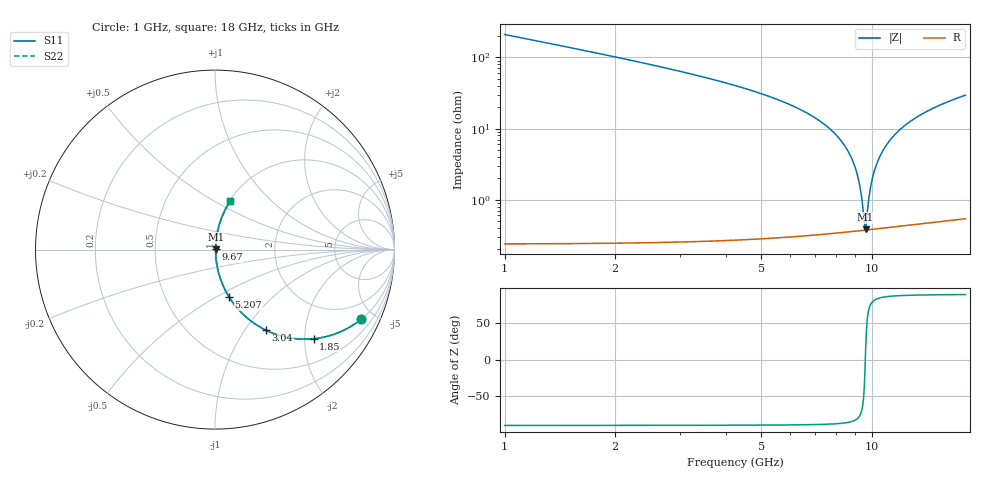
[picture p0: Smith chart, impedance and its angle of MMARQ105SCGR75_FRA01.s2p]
! MMARQ105SCGR75_FRA01  S-PARAMETER MODEL  ( General Type )
! Model Generated by TAIYO YUDEN Corporation (http://www.ty-top.com)
! Version 1.0
! TAIYO YUDEN Control No. 200326
! Copyright(c) 2020 TAIYO YUDEN CO.,LTD. All Rights Reserved.
! Product Description (link to TY-COMPAS)
! https://ds.yuden.co.jp/TYCOMPAS/or/detail?pn=MMARQ105SCGR75BFRA01&u=M
! Products Name : Multilayer Ceramic Capacitors
! Characteristics :
!  Capacitance : 0.75 pF , Rated Voltage : 250V , TCC : CG / C0G
!  Case Size : 1.0 x 0.5 / 0.039 x 0.02 [mm/inch] , Thickness : 0.5 / 0.02 [mm/inch]
!  (Conditions: Temperature = 25 degC , DC Bias Current/Voltage = 0A / 0V)
! External Node Assignments :
!  1  o---| |---o  2
! GND o---------o GND
! Frequency Range : 1GHz  -  18GHz  [ 401 STEP ]
# MHz S RI R 50
! Freq[MHz].  S11 Real  S11 Imag  S21 Real  S21 Imag  S12 Real  S12 Imag  S22 Real  S22 Imag
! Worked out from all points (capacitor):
!   401 points, 1 GHz to 18 GHz, reference 50 ohm
!   read as one part in series: C = 750 fF near 1.085 GHz
!   lowest |Z| = 384 mohm at 9.627 GHz (marker M1)
!   series resonance near 9.608 GHz, so ESL is about 370 pH
!   S11 on the Smith chart (normalised r, x): 1 GHz: 1.00, -4.20; 1.85 GHz: 1.00, -2.21; 3.04 GHz: 1.01, -1.26; 5.207 GHz: 1.01, -0.58; 9.67 GHz: 1.01, +0.01; 18 GHz: 1.01, +0.59
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1000  0.8148 -0.3879  0.1852 0.3879  0.1852 0.3879  0.8148 -0.3879
1850  0.5494 -0.4965  0.4506 0.4965  0.4506 0.4965  0.5494 -0.4965
3040  0.2836 -0.4487  0.7164 0.4487  0.7164 0.4487  0.2836 -0.4487
3847.5  0.1779 -0.3796  0.8221 0.3796  0.8221 0.3796  0.1779 -0.3796
5207.5  0.0786 -0.2642  0.9214 0.2642  0.9214 0.2642  0.0786 -0.2642
6695  0.0287 -0.1577  0.9713 0.1577  0.9713 0.1577  0.0287 -0.1577
7885  0.0109 -0.0865  0.9891 0.0865  0.9891 0.0865  0.0109 -0.0865
8692.5  0.00545 -0.0438  0.9946 0.0438  0.9946 0.0438  0.00545 -0.0438
9202.5  0.00398 -0.0189  0.996 0.0189  0.996 0.0189  0.00398 -0.0189
9372.5  0.00378 -0.0109  0.9962 0.0109  0.9962 0.0109  0.00378 -0.0109
9500  0.00372 -0.00495  0.9963 0.00495  0.9963 0.00495  0.00372 -0.00495
9585  0.00371 -0.00106  0.9963 0.00106  0.9963 0.00106  0.00371 -0.00106
9627.5  0.00372 0.000879  0.9963 -0.000879  0.9963 -0.000879  0.00372 0.000879
9670  0.00374 0.0028  0.9963 -0.0028  0.9963 -0.0028  0.00374 0.0028
9840  0.00387 0.0104  0.9961 -0.0104  0.9961 -0.0104  0.00387 0.0104
9967.5  0.00405 0.0161  0.9959 -0.0161  0.9959 -0.0161  0.00405 0.0161
10180  0.00448 0.0253  0.9955 -0.0253  0.9955 -0.0253  0.00448 0.0253
10435  0.0052 0.0361  0.9948 -0.0361  0.9948 -0.0361  0.0052 0.0361
11200  0.00857 0.0669  0.9914 -0.0669  0.9914 -0.0669  0.00857 0.0669
12347.5  0.0164 0.1092  0.9836 -0.1092  0.9836 -0.1092  0.0164 0.1092
15195  0.046 0.1981  0.954 -0.1981  0.954 -0.1981  0.046 0.1981
18000  0.0838 0.2681  0.9162 -0.2681  0.9162 -0.2681  0.0838 0.2681
